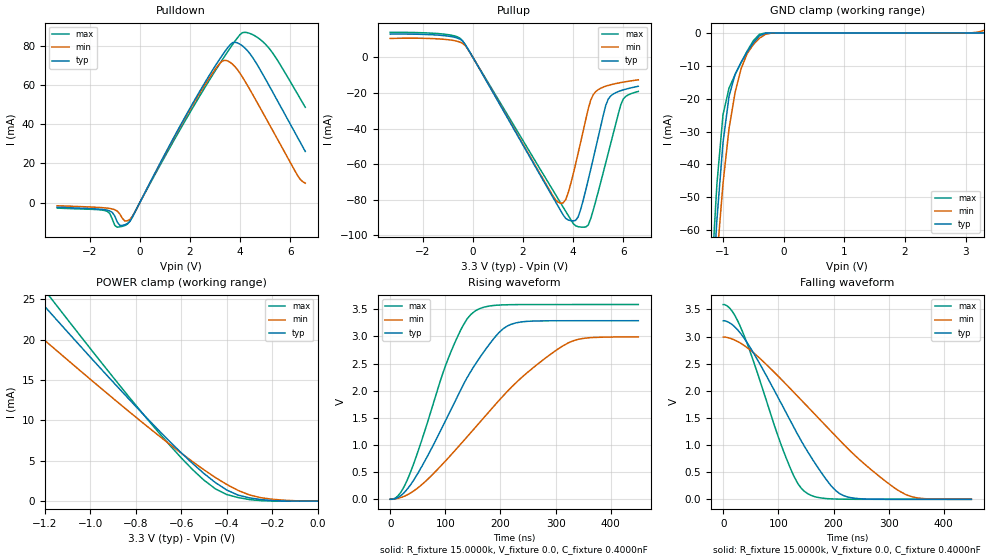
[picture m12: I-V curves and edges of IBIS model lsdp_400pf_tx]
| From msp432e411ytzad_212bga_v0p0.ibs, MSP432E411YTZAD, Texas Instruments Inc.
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|   Model lsdp_400pf_tx
[Model]		lsdp_400pf_tx
Model_type	3-state
Polarity   Non-Inverting
Enable   Active-Low
C_comp   7.0000pF   7.0000pF   7.0000pF
[Model Spec]
Vmeas 1.65 1.5 1.8
[Temperature Range]	  27.0000   0.1250k   -40.0000
[Voltage Range]   3.3000V   3.0000V   3.6000V
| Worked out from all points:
|   slope of the pulldown table from 0 to 0.495 V, typ, clamps not added: 39.8 ohm
|   slope of the pullup table from 0 to 0.495 V, typ, clamps not added: 40.7 ohm
|   GND clamp passes 1 mA (typ) near -0.40 V on its own axis
|   POWER clamp passes 1 mA (typ) near -0.37 V on its own axis
|   rising waveform, R_fixture 15.0000k, V_fixture 0.0, C_fixture 0.4000nF: 20-80 % time 104ns typ, 165ns min, 71.8ns max; typ from 0 V to 3.29 V
|   falling waveform, R_fixture 15.0000k, V_fixture 0.0, C_fixture 0.4000nF: 20-80 % time 108ns typ, 175ns min, 72.6ns max; typ from 3.29 V to 0 V
[Pulldown]
|Voltage	  I(typ)   I(min)   I(max)
-3.3V     -2.401mA   -1.67mA    -2.857mA
-1.4V     -3.695mA   -2.753mA   -4.133mA
-900mV    -10.07mA   -4.442mA   -12.64mA
-600mV    -11.42mA   -9.457mA   -11.81mA
-400mV    -9.699mA   -8.629mA   -9.649mA
2.3V      55.06mA    54.16mA    52.67mA
3.4V      77.55mA    72.9mA     75.3mA
3.9V      81.79mA    67.98mA    84.5mA
4.2V      79.09mA    62.05mA    87.23mA
4.7V      70.25mA    50.81mA    84.54mA
5.3V      56.6mA     36.92mA    76.61mA
6.6V      26.2mA     9.903mA    48.81mA
[Pullup]
|Voltage	  I(typ)   I(min)   I(max)
-3.3V     13.1mA     10.64mA    14.09mA
-500mV    10.12mA    8.492mA    10.61mA
-100mV    2.446mA    2.373mA    2.323mA
3.3V      -81.22mA   -80.03mA   -77.15mA
3.7V      -90.41mA   -79.99mA   -86.42mA
4.2V      -89.61mA   -53.77mA   -95.13mA
4.5V      -74.71mA   -35.11mA   -95.31mA
4.7V      -62.98mA   -24.03mA   -90.63mA
4.9V      -50.92mA   -19.26mA   -80.83mA
5.4V      -23.44mA   -15.74mA   -53.79mA
6V        -18.25mA   -13.89mA   -23.35mA
6.6V      -16.21mA   -12.59mA   -19.12mA
[GND_clamp]
|Voltage	  I(typ)   I(min)   I(max)
-3.3V     -840.3mA   -734.3mA   -920.6mA
-1.2V     -86.68mA   -94.57mA   -77.88mA
-1.1V     -56.77mA   -68.53mA   -45.9mA
-1V       -33.38mA   -45.87mA   -24.89mA
-900mV    -19.23mA   -29mA      -16.73mA
-800mV    -12.52mA   -18.04mA   -12.67mA
-700mV    -8.862mA   -10.78mA   -8.95mA
-600mV    -5.755mA   -6.231mA   -5.45mA
-400mV    -896.9uA   -1.614mA   -397.4uA
-200mV    -8.59uA    -49.41uA   -5.163uA
3V        2.546uA    8.612uA    1.975uA
3.3V      3.54uA     771.7uA    2.816uA
[POWER_clamp]
|Voltage	  I(typ)   I(min)   I(max)
-3.3V     110.9mA    96.85mA    135.1mA
-1.4V     30.43mA    24.76mA    33.43mA
-1.25V    25.67mA    21.1mA     27.93mA
-1.2V     24.09mA    19.89mA    26.11mA
-1.15V    22.51mA    18.68mA    24.29mA
-900mV    14.75mA    12.73mA    15.35mA
-700mV    8.795mA    8.133mA    8.526mA
-550mV    4.663mA    4.89mA     3.906mA
-450mV    2.303mA    2.932mA    1.531mA
-350mV    747.8uA    1.329mA    444.6uA
-250mV    199.2uA    426.7uA    62.4uA
0V        3.54uA     8.612uA    3.643uA
[Ramp]
| variable   typ   min   max
dV/dt_r		1.9746/98.5463n   1.7950/0.1600u   2.1537/65.0865n
dV/dt_f		1.9747/0.1006u   1.7952/0.1645u   2.1539/65.1122n
R_load =	15.0000k
[Rising Waveform]
R_fixture=	15.0000k
V_fixture=	0.0
V_fixture_min=	0.0
V_fixture_max=	0.0
C_fixture=	0.4000nF
|time   V(typ)   V(min)   V(max)
0s        63.74uV    44.73uV    95.15uV
14.86ns   38.7mV     18.98mV    73.05mV
30.63ns   183.9mV    79.89mV    348.9mV
105.4ns   1.555V     763.1mV    2.598V
131.5ns   2.093V     1.06V      3.191V
149.5ns   2.411V     1.268V     3.435V
190.5ns   2.994V     1.744V     3.574V
213.5ns   3.199V     2V         3.585V
318ns     3.291V     2.856V     3.59V
450ns     3.291V     2.991V     3.59V
[Falling Waveform]
R_fixture=	15.0000k
V_fixture=	0.0
V_fixture_min=	0.0
V_fixture_max=	0.0
C_fixture=	0.4000nF
|time   V(typ)   V(min)   V(max)
0s        3.291V     2.992V     3.59V
14.41ns   3.235V     2.962V     3.49V
31.53ns   3.058V     2.878V     3.171V
112.6ns   1.624V     2.135V     801.6mV
132.4ns   1.245V     1.926V     340.5mV
148.6ns   953.2mV    1.754V     135.3mV
195.9ns   246.1mV    1.25V      8.258mV
223.4ns   50.27mV    961.6mV    1.677mV
332.4ns   112.3uV    82.06mV    97.42uV
450ns     63.72uV    106.8uV    95.23uV
